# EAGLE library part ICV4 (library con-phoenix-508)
PHOENIX
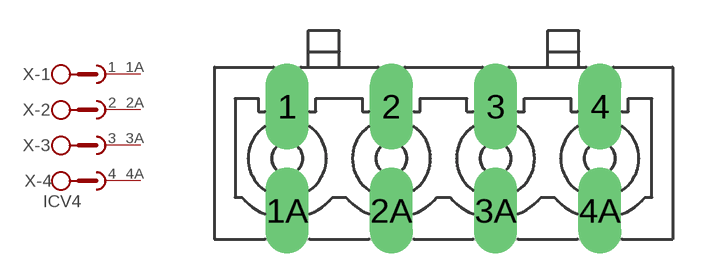
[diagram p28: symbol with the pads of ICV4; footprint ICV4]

Designator prefix X; gates -1=SKB2 -2=SKB2 -3=SKB2 -4=SKB2V

## ICV4 (OC_FARNELL: unknown; OC_NEWARK: unknown)  [ICV4]
1  -1:1  pas
1A  -1:2  pas
2  -2:1  pas
2A  -2:2  pas
3  -3:1  pas
3A  -3:2  pas
4  -4:1  pas
4A  -4:2  pas

## Footprint ICV4 (pad centres in mm)
PHOENIX
drill 1.397 long: 1 -7.62,2.54; 1A -7.62,-2.54; 2 -2.54,2.54; 2A -2.54,-2.54; 3 2.54,2.54; 3A 2.54,-2.54; 4 7.62,2.54; 4A 7.62,-2.54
